(* Logix 5000 Rung export; software revision 36.00 *)

VAR_GLOBAL   (* controller tags *)
   ISDU_Path : STRING[8] := ([0] := '$13$p192.168.0.50$04$00', [1] := '$13$p192.168.0.50$04$02', [2] := '$13$p192.168.0.50$04$04', [3] := '$13$p192.168.0.50$04$06', [4] := '$13$p192.168.0.50$04$08', [5] := '$13$p192.168.0.50$04$l', [6] := '$13$p192.168.0.50$04$p', [7] := '$13$p192.168.0.50$04$0E');
END_VAR

PROGRAM MainProgram

ROUTINE MainRoutine   (* ladder *)
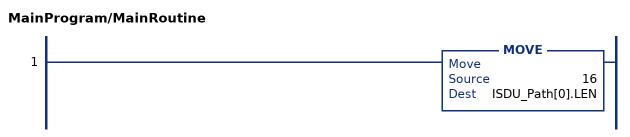
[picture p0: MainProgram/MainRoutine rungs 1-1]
   1: MOVE(16,ISDU_Path[0].LEN);
END_ROUTINE
END_PROGRAM
